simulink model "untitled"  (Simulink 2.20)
settings: Solver=ode45  StartTime=0.0  StopTime=50.0  RelTol=1e-3  AbsTol=1e-6

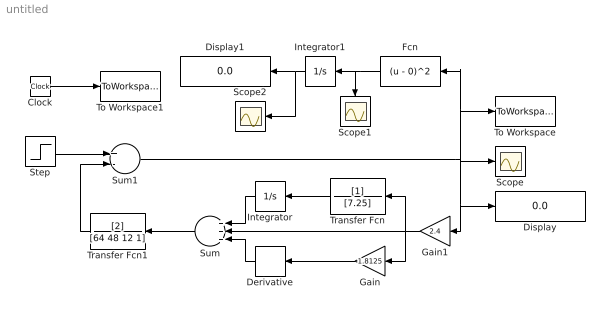
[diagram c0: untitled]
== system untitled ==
  Clock : Clock
  Derivative : Derivative  Orientation=left
  Display : Display
  Display1 : Display
  Fcn : Fcn  Orientation=left  Expr=(u - 0)^2
  Gain : Gain  Orientation=left  Gain=1.8125
  Gain1 : Gain  Orientation=left  Gain=2.4
  Integrator : Integrator  Orientation=left  ExternalReset=none  InitialConditionSource=internal  InitialCondition=0  LimitOutput=off  UpperSaturationLimit=inf  LowerSaturationLimit=-inf  ShowSaturationPort=off  ShowStatePort=off  AbsoluteTolerance=auto
  Integrator1 : Integrator  Orientation=left  ExternalReset=none  InitialConditionSource=internal  InitialCondition=0  LimitOutput=off  UpperSaturationLimit=inf  LowerSaturationLimit=-inf  ShowSaturationPort=off  ShowStatePort=off  AbsoluteTolerance=auto
  Scope : Scope
  Scope1 : Scope
  Scope2 : Scope
  Step : Step  Time=0  Before=0  After=1
  Sum : Sum  Orientation=left  Inputs=+++
  Sum1 : Sum  Inputs=+-
  To Workspace : ToWorkspace  VariableName=d  SampleTime=-1
  To Workspace1 : ToWorkspace  VariableName=t  SampleTime=-1
  Transfer Fcn : TransferFcn  Orientation=left  Numerator=[1]  Denominator=[7.25]
  Transfer Fcn1 : TransferFcn  Orientation=left  Numerator=[2]  Denominator=[64 48 12 1]
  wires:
  Transfer Fcn/1 -> Integrator/1
  Gain/1 -> Derivative/1
  Derivative/1 -> Sum/3
  Integrator/1 -> Sum/1
  Sum/1 -> Transfer Fcn1/1
  Gain1/1 -> Sum/2, Transfer Fcn/1, Gain/1
  Transfer Fcn1/1 -> Sum1/2
  Step/1 -> Sum1/1
  Clock/1 -> To Workspace1/1
  Sum1/1 -> Scope/1, To Workspace/1, Fcn/1, Gain1/1, Display/1
  Integrator1/1 -> Display1/1, Scope2/1
  Fcn/1 -> Integrator1/1, Scope1/1
